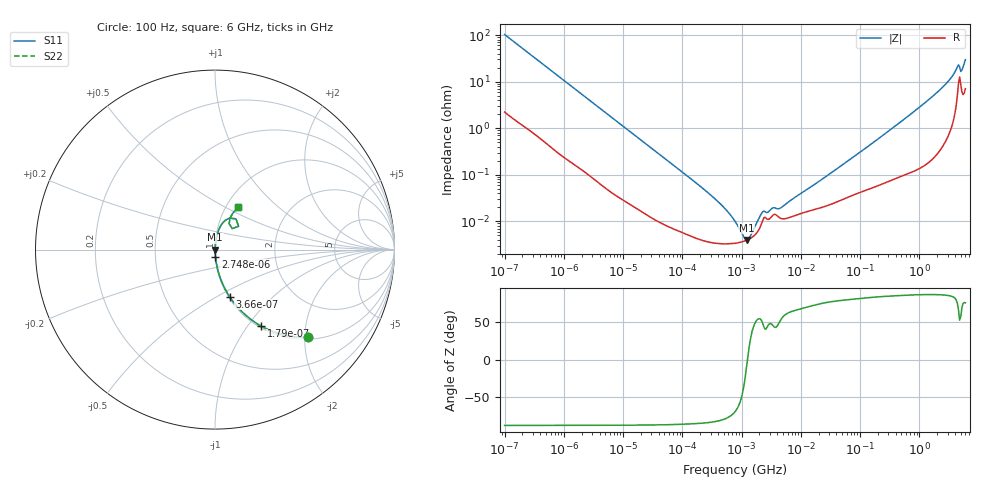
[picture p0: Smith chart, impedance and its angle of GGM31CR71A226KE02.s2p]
!Murata Part Number: GGM31CR71A226KE02
!These Parameters are Measured in Series Mode Connection
!Data Generated on Mar 13, 2026
!  o--ll--o
!Port1  Port2
!  o------o
!Operation Temp=25[degC], DC Bias Voltage=0[V]
!Freq. Start=100[Hz] Stop=6[GHz] 401[Steps]
# Hz S RI R 50
!Freq.(Hz) S11(Real) S11(Imag) S21(Real) S21(Imag) S12(Real) S12(Imag) S22(Real) S22(Imag)
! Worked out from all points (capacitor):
!   401 points, 100 Hz to 6 GHz, reference 50 ohm
!   read as one part in series: C = 15.3 uF near 109 Hz
!   lowest |Z| = 3.97 mohm at 1.212 MHz (marker M1)
!   series resonance near 1.258 MHz, so ESL is about 1 nH
!   S11 on the Smith chart (normalised r, x): 100 Hz: 1.04, -2.07; 179 Hz: 1.03, -1.16; 366 Hz: 1.01, -0.58; 2.748 kHz: 1.00, -0.08; 6 GHz: 1.14, +0.58
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100  0.5168 -0.4891  0.4832 0.4891  0.4832 0.4891  0.5168 -0.4891
179  0.2579 -0.4267  0.7421 0.4267  0.7421 0.4267  0.2579 -0.4267
366  0.0815 -0.2624  0.9185 0.2624  0.9185 0.2624  0.0815 -0.2624
784  0.0209 -0.1325  0.9791 0.1325  0.9791 0.1325  0.0209 -0.1325
2008  0.00414 -0.0534  0.9959 0.0534  0.9959 0.0534  0.00414 -0.0534
2748  0.00249 -0.0393  0.9975 0.0393  0.9975 0.0393  0.00249 -0.0393
40335  0.000104 -0.00279  0.9999 0.00279  0.9999 0.00279  0.000104 -0.00279
302498  3.52e-05 -0.000364  1 0.000364  1 0.000364  3.52e-05 -0.000364
495019  3.28e-05 -0.0002  1 0.0002  1 0.0002  3.28e-05 -0.0002
774597  3.37e-05 -9.47e-05  1 9.47e-05  1 9.47e-05  3.37e-05 -9.47e-05
1212075  3.91e-05 -7.1e-06  1 7.1e-06  1 7.1e-06  3.91e-05 -7.1e-06
1734173  5.32e-05 6.53e-05  0.9999 -6.53e-05  0.9999 -6.53e-05  5.32e-05 6.53e-05
2372521  0.000119 0.000116  0.9999 -0.000116  0.9999 -0.000116  0.000119 0.000116
3394479  0.000136 0.000139  0.9999 -0.000139  0.9999 -0.000139  0.000136 0.000139
4643984  0.000115 0.000159  0.9999 -0.000159  0.9999 -0.000159  0.000115 0.000159
1.555665e7  0.000174 0.000547  0.9998 -0.000547  0.9998 -0.000547  0.000174 0.000547
3.124326e8  0.00081 0.00892  0.9992 -0.00892  0.9992 -0.00892  0.00081 0.00892
1.873145e9  0.00548 0.0543  0.9945 -0.0543  0.9945 -0.0543  0.00548 0.0543
3.065283e9  0.0166 0.0988  0.9834 -0.0988  0.9834 -0.0988  0.0166 0.0988
4.193612e9  0.0583 0.1639  0.9417 -0.1639  0.9417 -0.1639  0.0583 0.1639
5.245841e9  0.0789 0.144  0.9211 -0.144  0.9211 -0.144  0.0789 0.144
6e9  0.1293 0.2349  0.8707 -0.2349  0.8707 -0.2349  0.1293 0.2349
